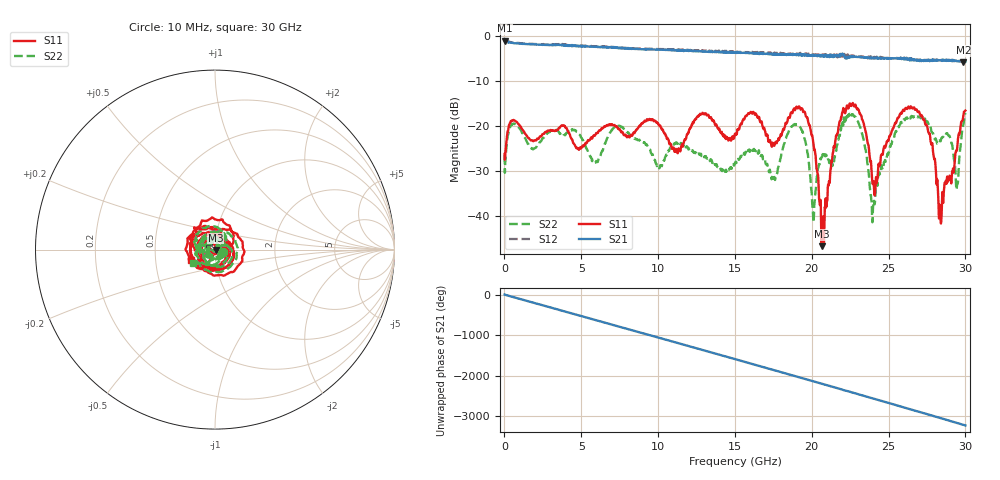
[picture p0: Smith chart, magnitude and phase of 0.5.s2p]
!Agilent Technologies,E8364B,US42250130,A.04.87.01
!Agilent E8364B: A.04.87.01
!Date: Monday, February 07, 2022 23:47:47
!Correction: S11(Full 2 Port SOLT,1,2) S21(Full 2 Port SOLT,1,2) S12(Full 2 Port SOLT,1,2) S22(Full 2 Port SOLT,1,2)
!S2P File: Measurements: S11, S21, S12, S22:
# Hz S  dB  R 50
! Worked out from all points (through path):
!   1601 points, 10 MHz to 30 GHz, reference 50 ohm
!   highest |S21| = -1.02 dB at 28.74 MHz (marker M1); lowest = -5.8 dB at 29.87 GHz (marker M2)
!   group delay of S21, straight-line fit = 298 ps
!   lowest |S11| = -46.8 dB at 20.65 GHz (marker M3), VSWR 1.01, Z = 50.4 - j0.279 ohm
!   |S11| at or under -10 dB: start of sweep to end of sweep
!   |S22| runs from -41.4 to -17.1 dB; largest |S21 - S12| = 0.085
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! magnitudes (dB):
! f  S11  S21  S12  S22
! 10 MHz  -26.2  -1.0  -1.1  -26.6
! 28.74 MHz  -27.5  -1.0  -1.0  -30.4
! 553.6 MHz  -18.7  -1.5  -1.4  -19.6
! 5.015 GHz  -24.8  -2.2  -2.1  -22.6
! 5.952 GHz  -21.7  -2.4  -2.2  -28.0
! 7.564 GHz  -21.1  -2.7  -2.6  -20.1
! 10.02 GHz  -19.6  -3.0  -2.9  -29.0
! 15.01 GHz  -21.7  -3.6  -3.6  -28.3
! 16.13 GHz  -17.1  -3.7  -3.5  -25.4
! 17.54 GHz  -24.3  -4.0  -4.0  -32.2
! 19.03 GHz  -15.8  -4.1  -3.9  -19.6
! 20.01 GHz  -22.0  -4.2  -4.0  -35.7
! 20.65 GHz  -46.8  -4.3  -4.3  -26.9
! 22.17 GHz  -17.2  -4.8  -4.2  -18.2
! 23.16 GHz  -17.3  -4.7  -4.7  -20.3
! 23.98 GHz  -32.9  -4.9  -4.6  -38.4
! 25.01 GHz  -22.9  -5.0  -4.9  -25.8
! 27.08 GHz  -17.5  -5.2  -5.4  -18.2
! 28.41 GHz  -41.7  -5.3  -5.4  -23.2
! 29.44 GHz  -25.4  -5.5  -5.6  -33.9
! 29.87 GHz  -17.7  -5.8  -5.4  -19.7
! 30 GHz  -16.6  -5.6  -5.7  -17.1
